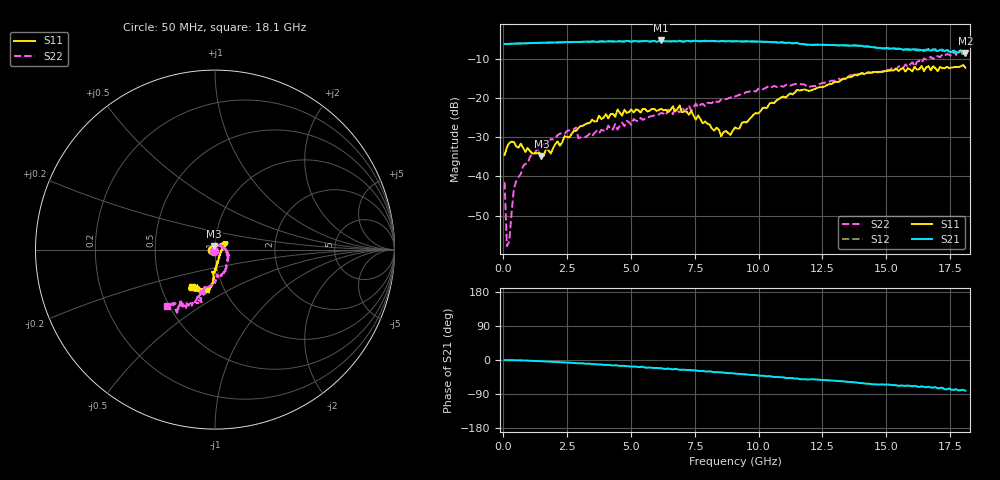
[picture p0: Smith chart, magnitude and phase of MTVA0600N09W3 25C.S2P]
! Network Analyzer HP8720D.06.14 Serial No. US36140669
! 10 May 2005  14:40:38
! Frequency  S11  S21  S12  S22
# HZ  S  DB R 50
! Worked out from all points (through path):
!   201 points, 50 MHz to 18.1 GHz, reference 50 ohm
!   highest |S21| = -5.24 dB at 6.187 GHz (marker M1); lowest = -8.5 dB at 18.1 GHz (marker M2)
!   group delay of S21, straight-line fit = 12.8 ps
!   lowest |S11| = -34.8 dB at 1.494 GHz (marker M3), VSWR 1.04, Z = 49.5 + j1.74 ohm
!   |S11| at or under -10 dB: start of sweep to end of sweep
!   |S22| runs from -57.8 to -7.7 dB; largest |S21 - S12| = 0.022
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5e7  -34.49 -173.2  -6.14 -0.3  -6.16 -0.5  -41.49 -121.7
1.4025e8  -32.56 178.6  -6.14 -0.3  -6.16 -0.7  -57.80 124.8
2.305e8  -31.44 171.4  -6.12 -0.2  -6.10 -0.7  -56.59 96.2
4.11e8  -31.17 166.0  -6.06 -0.6  -6.07 -1.0  -43.18 99.6
5.0125e8  -32.27 165.2  -6.07 -0.7  -6.04 -1.0  -41.19 79.7
1.494e9  -34.77 105.8  -5.85 -3.4  -5.84 -3.7  -32.33 56.1
2.84775e9  -28.34 46.8  -5.62 -8.3  -5.60 -8.5  -27.49 41.5
2.938e9  -27.64 45.3  -5.65 -8.8  -5.61 -9.1  -30.20 48.5
3.1185e9  -27.06 43.6  -5.57 -8.8  -5.59 -9.4  -29.90 42.0
4.382e9  -24.75 34.3  -5.48 -13.8  -5.51 -14.8  -26.60 23.0
4.47225e9  -22.86 32.1  -5.51 -14.5  -5.40 -14.7  -28.02 22.9
4.65275e9  -24.46 30.2  -5.51 -15.2  -5.47 -16.2  -26.25 23.0
4.743e9  -22.92 34.3  -5.55 -15.7  -5.46 -15.8  -27.16 16.4
6.09675e9  -22.99 29.3  -5.43 -21.6  -5.37 -22.1  -24.15 -0.6
6.187e9  -22.69 32.2  -5.24 -21.7  -5.28 -22.3  -23.72 -5.6
6.909e9  -21.86 28.7  -5.35 -26.0  -5.33 -25.8  -23.61 -18.6
8.5335e9  -29.68 -10.6  -5.40 -33.0  -5.41 -33.5  -20.33 -43.3
9.075e9  -27.46 -45.2  -5.44 -35.8  -5.43 -36.3  -19.56 -51.9
1.088e10  -19.82 -86.9  -5.70 -45.7  -5.75 -46.4  -16.89 -72.8
1.21435e10  -17.79 -93.7  -6.39 -50.8  -6.36 -51.5  -16.89 -83.7
1.512175e10  -12.81 -99.1  -7.32 -65.0  -7.31 -65.9  -13.05 -103.4
1.81e10  -12.19 -121.3  -8.51 -81.2  -8.18 -82.5  -7.75 -130.2
